(* IEC 60870-5-101 system configuration parameter *)
TYPE ST_IEC870_5_101SSysPara :
STRUCT
	asduAddr	: WORD := 1;(* Common address of ASDU *)

	nOrg		: BYTE := 0;(* Originator address *)

	
	asduFmt		: ST_IEC870_5_101AsduFmtParams := ( eCOTSize := eIEC870_COT_OneOctet,
													eAsduAddrSize := eIEC870_AsduAddr_OneOctet,
													eObjAddrSize := eIEC870_ObjAddr_TwoOctets );(* ASDU frame format parameter (octet lengths) *)

	bCoro		: BOOL := FALSE;(* Enable/disable local counter freeze/reset command *)
	eCoroMode	: E_IEC870_5_101CoroMode := eIEC870_CoroMode_A;(* Counter interrogation operation mode *)
	bCoroReset	: BOOL := FALSE;(* TRUE => Enable local reset of counter values *)
	tCoro		: TIME := T#60S;(* Local freeze and reset cycle *)										
														
	bCyclic		: BOOL := FALSE;(* TRUE => Send cyclic data *)
	tCyclic		: TIME := T#60s;(* Cycle time of cyclic data *)														

	bDbgLink 	: BOOL := FALSE;(* TRUE => Log serial link layer frames to TwinCAT output window *)
	bDbgAppl 	: BOOL := FALSE;(* TRUE => Log application layer messages immediatelly to TwinCAT output window *)
	eDbgAsdu 	: E_IEC870_5_101FifoDbgFlags := eIEC870_FIFO_DBG_OFF;(* eIEC870_FIFO_DBG_ALL => Log ASDU TX/RX fifo frames to TwinCAT output window *)
END_STRUCT
END_TYPE
